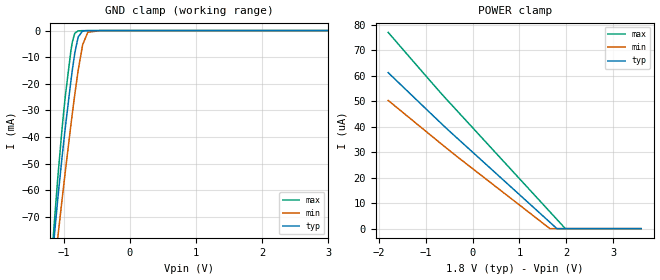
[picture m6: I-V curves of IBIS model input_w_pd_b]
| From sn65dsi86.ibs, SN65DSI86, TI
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|   Model
[Model]   input_w_pd_b
Model_type   Input
Vinl = 0.54
Vinh = 1.26
|   typ   min   max
C_comp   1.129pF   1.082pF   1.175pF
[Voltage Range]   1.8   1.65   1.98
[Temperature Range]   27   125   -40
[Power Clamp Reference]   1.8   1.65   1.98
[GND Clamp Reference]   -0   -0   -0
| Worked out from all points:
|   GND clamp passes 1 mA (typ) near -0.74 V on its own axis
[GND Clamp]
|   Voltage   I(typ)   I(min)   I(max)
-1.8V     -308mA     -294.7mA   -317.4mA
-1.217V   -100.4mA   -108.5mA   -98.83mA
-1.141V   -77.88mA   -90.31mA   -72.91mA
-1.087V   -63.43mA   -77.99mA   -55.6mA
-968.4mV  -35.54mA   -52.06mA   -23.67mA
-865.8mV  -14.63mA   -30.96mA   -4.213mA
-828mV    -8.23mA    -23.69mA   -978uA
-779.4mV  -2.443mA   -15.05mA   -117.5uA
-709.2mV  -147.3uA   -5.196mA   -18.6uA
-633.6mV  -14.93uA   -651.5uA   -12.8uA
-450mV    -7.495uA   -7.246uA   -8.993uA
3.595V    0A         0A         0A
[POWER Clamp]
|   Voltage   I(typ)   I(min)   I(max)
-1.8V     61.17uA    50.27uA    76.95uA
-628.2mV  40.54uA    32.64uA    52.16uA
1.645V    2.572uA    59.87nA    6.688uA
1.796V    52.22nA    0A         3.664uA
1.975V    0A         0A         100.9nA
3.595V    0A         0A         0A
